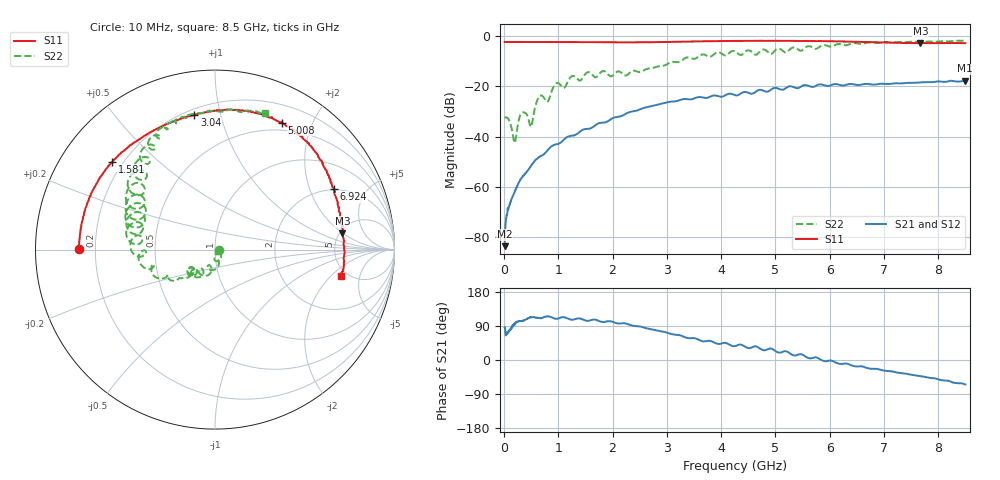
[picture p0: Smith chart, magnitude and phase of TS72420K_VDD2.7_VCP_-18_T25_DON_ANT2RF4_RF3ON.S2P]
!Agilent Technologies,E5071C,MY46417908,A.11.23
!Date: Thu Oct 03 16:41:31 2019
!Data & Calibration Information:
!Freq	S11:SOLT2(ON)	S21:SOLT2(ON)	S12:SOLT2(ON)	S22:SOLT2(ON)
!PortZ  Port1:50+j0  Port2:50+j0
!Above PortZ is port z conversion or system Z0 setting when saving the data.
!When reading, reference impedance value at option line is always used.
# Hz S dB R 50
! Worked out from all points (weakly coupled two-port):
!   1601 points, 10 MHz to 8.5 GHz, reference 50 ohm
!   highest |S21| = -17.81 dB at 8.484 GHz (marker M1); lowest = -83.6 dB at 10 MHz (marker M2)
!   lowest |S11| = -2.9 dB at 7.672 GHz (marker M3), VSWR 6.04, Z = 263 + j99 ohm
!   |S11| at or under -10 dB: nowhere
!   |S22| runs from -42.6 to -1.8 dB; largest |S21 - S12| = 0.0015
!   S11 on the Smith chart (normalised r, x): 10 MHz: 0.14, +0.00; 1.581 GHz: 0.16, +0.36; 3.04 GHz: 0.23, +0.83; 5.008 GHz: 0.40, +1.59; 6.924 GHz: 1.95, +2.97; 8.5 GHz: 4.39, -2.68
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1e7  -2.38 179.8  -83.59 86.2  -82.13 93.3  -32.61 -2.8
7.898125e7  -2.40 177.7  -68.67 73.5  -68.38 75.3  -32.95 -36.2
1.904125e8  -2.43 174.5  -62.35 91.6  -62.57 93.6  -42.49 -40.8
3.28375e8  -2.41 170.7  -56.28 103.4  -56.19 103.6  -30.45 -34.8
4.822562e8  -2.43 166.6  -52.17 113.1  -52.11 112.0  -35.91 -68.4
5.300125e8  -2.43 165.2  -50.74 113.0  -50.75 112.6  -33.13 -33.8
6.573625e8  -2.41 162.1  -47.96 110.3  -47.98 110.5  -23.86 -68.0
7.95325e8  -2.43 158.4  -45.65 115.2  -45.67 115.2  -26.25 -87.6
9.598188e8  -2.41 154.4  -43.06 108.9  -43.11 108.9  -18.81 -94.8
1.426769e9  -2.45 142.9  -37.60 108.3  -37.59 108.2  -17.34 -118.5
1.58065e9  -2.46 139.5  -36.85 104.3  -36.82 104.4  -14.49 -134.4
2.238625e9  -2.55 121.5  -31.00 96.5  -31.00 96.5  -15.80 -138.8
2.843538e9  -2.45 104.1  -27.28 76.9  -27.28 76.8  -12.11 -139.9
3.039869e9  -2.39 98.7  -26.22 70.4  -26.21 70.3  -10.81 -142.9
4.255e9  -1.98 74.7  -23.55 36.5  -23.54 36.5  -6.13 164.1
5.008488e9  -1.93 62.1  -20.66 22.8  -20.61 22.8  -5.47 157.6
5.671769e9  -2.06 51.2  -20.26 4.9  -20.18 5.2  -4.42 132.6
6.924044e9  -2.56 27.0  -19.02 -25.2  -19.05 -25.2  -2.67 112.4
7.088538e9  -2.69 23.9  -19.13 -29.5  -19.10 -29.0  -2.57 107.4
7.672225e9  -2.91 7.4  -18.48 -42.3  -18.47 -42.0  -2.33 95.9
8.484081e9  -2.88 -11.4  -17.81 -63.8  -17.86 -64.2  -1.85 70.3
8.5e9  -2.87 -11.9  -17.84 -64.6  -17.89 -65.1  -1.80 69.9
